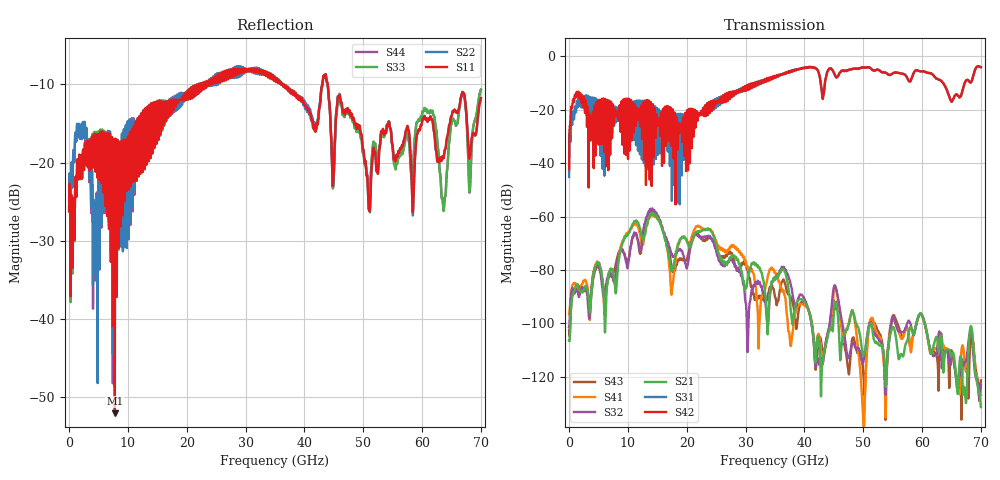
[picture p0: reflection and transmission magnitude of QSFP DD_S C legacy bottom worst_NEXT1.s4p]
! AWR Design Environment (8415) Thu Dec 20 15:41:23 2018
! Document = 'CHANNEL TEST'
! nPorts: 4, nXvals: 7001
# HZ S DB R 50
!Freq DBS11 AngS11 DBS12 AngS12 DBS13 AngS13 DBS14 AngS14
!	DBS21 AngS21 DBS22 AngS22 DBS23 AngS23 DBS24 AngS24
!	DBS31 AngS31 DBS32 AngS32 DBS33 AngS33 DBS34 AngS34
!	DBS41 AngS41 DBS42 AngS42 DBS43 AngS43 DBS44 AngS44
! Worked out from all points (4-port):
!   7000 points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, 10 MHz to 70 GHz, reference 50 ohm
!   strongest paths, dB at 10 MHz, 17.51 GHz, 35.01 GHz, 52.51 GHz, 70 GHz:
!     S42: -42.3, -23.4, -7.5, -5.0, -4.0
!     S31: -45.2, -30.1, -7.6, -5.0, -4.0
!     S21: -106.5, -80.2, -83.4, -107.4, -131.3
!     S32: -101.5, -74.2, -83.1, -105.5, -123.1
!     S41: -96.6, -87.2, -81.1, -104.5, -127.0
!     S43: -102.6, -78.9, -90.3, -102.7, -121.3
!   lowest |S11| = -52.1 dB at 7.78 GHz (marker M1), VSWR 1.00, Z = 49.9 - j0.242 ohm
!   |S11| at or under -10 dB: start of sweep to 21.78 GHz; 36.28 GHz to 43.07 GHz (6.789 GHz wide, 17.1 % of centre); 43.97 GHz to end of sweep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
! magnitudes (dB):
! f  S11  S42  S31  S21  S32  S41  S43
! 10 MHz  -26.3  -42.3  -45.2  -106.5  -101.5  -96.6  -102.6
! 1.3 GHz  -22.2  -13.3  -16.9  -85.7  -87.8  -86.1  -85.8
! 7.78 GHz  -52.1  -19.7  -18.9  -85.2  -83.7  -85.3  -79.5
! 14.08 GHz  -14.2  -25.5  -28.6  -58.6  -56.9  -58.8  -57.2
! 17.77 GHz  -12.9  -38.4  -30.8  -78.5  -74.8  -82.2  -80.3
! 21.93 GHz  -11.1  -22.1  -21.9  -65.4  -67.1  -63.4  -66.4
! 70 GHz  -11.8  -4.0  -4.0  -131.3  -123.1  -127.0  -121.3
